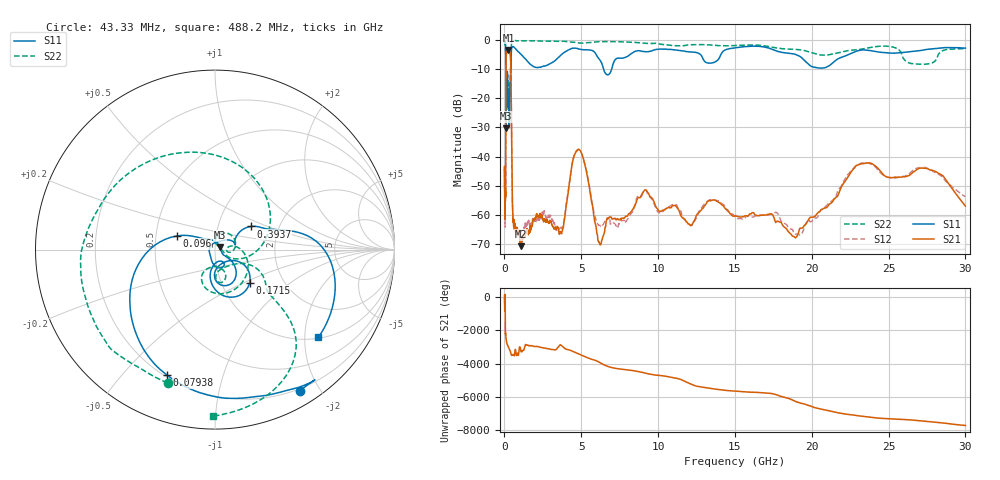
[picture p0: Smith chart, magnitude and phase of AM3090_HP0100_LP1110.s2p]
! Date/Time: Thu, Feb 28, 2019 1:58 PM
! Network Analyzer: Agilent Technologies E8364B Rev: A.07.50.67
! Sweep from 0.010 to 30.000 GHz, 1601 Points, Sweep Type: LOG
! Power Supply: 5.023 V, 0.002 A
# Hz S DB R 50
!freq MagS11 AngS11 MagS21 AngS21 MagS12 AngS12 MagS22 AngS22
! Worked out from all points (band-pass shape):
!   1601 points, 10 MHz to 30 GHz, reference 50 ohm
!   highest |S21| = -3.45 dB at 257.3 MHz (marker M1); lowest = -70.7 dB at 1.071 GHz (marker M2)
!   |S21| within 3 dB of the highest: 107.6 MHz to 396.7 MHz (289.1 MHz wide, 115 % of centre)
!   lowest |S11| = -30.4 dB at 103.5 MHz (marker M3), VSWR 1.06, Z = 52.8 + j1.43 ohm
!   |S11| at or under -10 dB: 94.45 MHz to 409.6 MHz (315.1 MHz wide, 125 % of centre); 6.454 GHz to 6.977 GHz (522.4 MHz wide, 7.78 % of centre)
!   |S22| runs from -31.5 to -0.2 dB; largest |S21 - S12| = 0.012
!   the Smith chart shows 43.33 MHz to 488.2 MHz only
!   S11 on the Smith chart (normalised r, x): 43.33 MHz: 0.18, -1.76; 79.38 MHz: 0.21, -0.67; 96 MHz: 0.64, +0.10; 171.5 MHz: 1.36, -0.54; 393.7 MHz: 1.44, +0.39; 488.2 MHz: 1.02, -2.33
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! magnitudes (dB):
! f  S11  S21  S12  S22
! 10 MHz  -0.2  -44.4  -45.2  -0.8
! 38.04 MHz  -0.5  -60.2  -58.4  -1.7
! 43.33 MHz  -0.8  -58.1  -62.6  -2.1
! 79.38 MHz  -2.5  -47.4  -47.4  -4.6
! 96 MHz  -12.9  -14.8  -14.8  -13.4
! 103.5 MHz  -30.4  -7.8  -7.8  -31.0
! 144.7 MHz  -20.9  -3.8  -3.7  -23.8
! 171.5 MHz  -11.5  -3.6  -3.6  -14.2
! 257.3 MHz  -21.7  -3.5  -3.4  -18.4
! 314.3 MHz  -30.1  -3.8  -3.8  -15.8
! 393.7 MHz  -12.5  -6.2  -6.2  -10.3
! 488.2 MHz  -2.4  -44.5  -45.0  -0.7
! 550.5 MHz  -2.4  -60.4  -59.4  -0.4
! 1.071 GHz  -4.9  -70.7  -66.2  -0.3
! 2.084 GHz  -9.5  -59.8  -61.4  -0.3
! 3.686 GHz  -5.2  -66.1  -64.2  -0.5
! 4.805 GHz  -3.1  -37.6  -37.5  -1.0
! 6.171 GHz  -6.6  -69.4  -63.6  -0.6
! 7.926 GHz  -5.9  -60.4  -62.0  -0.7
! 18.93 GHz  -5.0  -67.9  -66.7  -3.2
! 23.48 GHz  -3.5  -42.3  -42.2  -2.9
! 30 GHz  -2.8  -57.0  -53.7  -3.0
